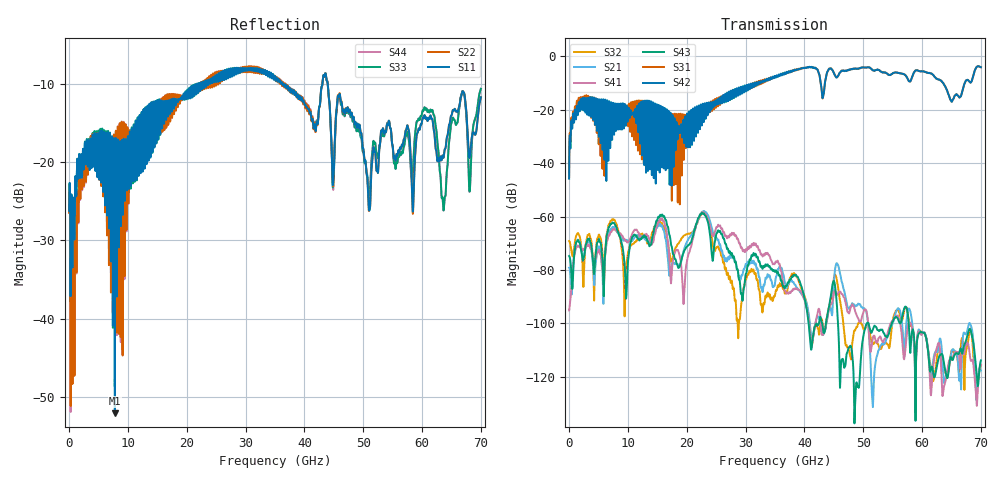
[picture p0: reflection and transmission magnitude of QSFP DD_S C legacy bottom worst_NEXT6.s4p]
! AWR Design Environment (8415) Thu Dec 20 15:48:25 2018
! Document = 'CHANNEL TEST'
! nPorts: 4, nXvals: 7001
# HZ S DB R 50
!Freq DBS11 AngS11 DBS12 AngS12 DBS13 AngS13 DBS14 AngS14
!	DBS21 AngS21 DBS22 AngS22 DBS23 AngS23 DBS24 AngS24
!	DBS31 AngS31 DBS32 AngS32 DBS33 AngS33 DBS34 AngS34
!	DBS41 AngS41 DBS42 AngS42 DBS43 AngS43 DBS44 AngS44
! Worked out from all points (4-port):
!   7000 points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, 10 MHz to 70 GHz, reference 50 ohm
!   strongest paths, dB at 10 MHz, 17.51 GHz, 35.01 GHz, 52.51 GHz, 70 GHz:
!     S42: -45.8, -24.5, -7.4, -5.0, -4.0
!     S31: -45.2, -30.1, -7.6, -5.0, -4.0
!     S43: -74.7, -71.9, -80.6, -102.5, -113.8
!     S41: -95.1, -79.3, -77.5, -106.2, -115.6
!     S21: -79.1, -77.4, -84.9, -110.7, -117.7
!     S32: -69.1, -76.1, -89.3, -107.8, -115.6
!   lowest |S11| = -52.1 dB at 7.78 GHz (marker M1), VSWR 1.00, Z = 49.9 - j0.242 ohm
!   |S11| at or under -10 dB: start of sweep to 21.78 GHz; 36.28 GHz to 43.07 GHz (6.789 GHz wide, 17.1 % of centre); 43.97 GHz to end of sweep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
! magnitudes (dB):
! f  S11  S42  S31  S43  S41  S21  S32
! 10 MHz  -26.3  -45.8  -45.2  -74.7  -95.1  -79.1  -69.1
! 1.65 GHz  -19.9  -17.1  -15.5  -69.4  -71.3  -69.2  -66.8
! 7.78 GHz  -52.1  -18.0  -18.9  -62.8  -64.8  -64.2  -61.5
! 9.49 GHz  -23.7  -17.9  -19.4  -79.5  -68.7  -69.0  -91.8
! 22.83 GHz  -9.8  -21.6  -19.5  -58.9  -58.5  -58.0  -58.6
! 27.05 GHz  -9.1  -16.7  -15.2  -72.3  -67.4  -75.5  -81.8
! 70 GHz  -11.8  -4.0  -4.0  -113.8  -115.6  -117.7  -115.6
